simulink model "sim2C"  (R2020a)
settings: Solver=ode15s  StartTime=0.0  StopTime=tsim  RelTol=1e-3
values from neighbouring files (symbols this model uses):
  d0 = 0    [run2C.m]    (also in Main.m = [Fh, Tcin, Thin]; Main_OL.m = [Fh, Tcin, Thin]; runTestCalcBlk.m = [Fh, Tcin, Thin]; runTransf.m = [Fh; Tcin; U0; Ffeed0; m0; Tfeed0])
  df = 0    [run2C.m]
  h0 = [LC1max ; LC1min; LC2max; LC2min; LC3max;LC3min ]    [run2C.m]
  hf = h0    [run2C.m]
  hmax = [2.3; 2.8; 3.2]    [run2C.m]
  Kc = 1./k.*1./(tauC+theta)    [run2C.m]    (also in Main.m = 1/k*tau/(tauC+theta); runTransf.m = 1/kM(i)*tau(i)/(tauCM(i)+theta(i)); runTransfOL.m = 1/kM(i)*tau(i)/(tauCM(i)+theta(i)))
  KI = Kc./tauI    [run2C.m]    (also in Main.m = Kp/tauIv; Main_OL.m = 1; runTransf.m = 1/kS(i)*1/tauCS(i); runTransfOL.m = 1/kS(i)*1/tauCS(i))
  nd = length(d0)    [run2C.m]    (also in Main.m = size(d0,2); Main_OL.m = size(d0,2); runTestCalcBlk.m = size(d0,2); runTransf.m = size(d0,1))
  np = length(param)    [run2C.m]    (also in runH2Psim.m; Main.m = size(p,2); Main_OL.m = size(p,2); runTestCalcBlk.m = size(p,2))
  nu = length(z0)    [run2C.m]    (also in runH2Psim.m = length(u0); Main.m = 1; Main_OL.m = 1; runTestCalcBlk.m = 1)
  nx = length(x0)    [run2C.m]    (also in H2P_Turbine_driven.m = param(end); runTD.m; H2P_Boiler_driven.m = param(end); runBD.m)
  param = [A; Cv; DP; rho; N]    [run2C.m]    (also in runTD.m = [Tref;TrefB;dHvap;cpg;cpW;cpSt;R;Mwt;     T0;TG0;ME;pC;     ; runBD.m = [Tref;TrefB;dHvap;cpg;cpW;cpSt;R;Mwt;          T0;TG0;ME;pC;; runFP.m = [Tref;TrefB;dHvap;cpg;cpW;cpSt;R;Mwt;          T0;TG0;ME;pC;; runFPV2.m = [Tref;TrefB;dHvap;cpg;cpW;cpSt;R;Mwt;          T0;TG0;ME;pC;)
  tauT = tauI./2    [run2C.m]
  td = 0    [run2C.m]
  th = ones(6,1)    [run2C.m]
  tz0OP = [10; tBend]    [run2C.m]
  tz1OP = [10; tBend]    [run2C.m]
  tz2OP = [10; tBend]    [run2C.m]
  tz3OP = [10; tBend]    [run2C.m]
  u0 = [z0(1); z0(2); z0(2); z0(3); z0(3); z0(4)]    [run2C.m]    (also in runH2Psim.m = [mG0;zV0;mP0;mB0;mA0]; calcblock.m = p(2); testfun.m = 5; u_function.m = 5)
  x0 = [hH; hH; hH].*hmax    [run2C.m]    (also in runTD.m = [TE0;TD0;TSh0;MD0; MSh0;w0;TA0;0;0;0;0;0;0;0;0;0]; runBD.m = [TE0;TD0;TSh0;MD0; MSh0;w0;TA0;0;0;0;0;0;0;0;0;0]; runFP.m = [TE0;TD0;TSh0;MD0; MSh0;w0;TA0;0;0;0;0;0;0;0]; runFPV2.m = [TE0;TD0;TSh0;MD0; MSh0;w0;TA0;0;0;0;0;0;0;0])
  zOP = z0.*[0.5; 1; 1; 1]    [run2C.m]
  zOP0 = [1;1;1;1]    [run2C.m]
undefined symbols (not defined in the file or in its folder): TanksODE

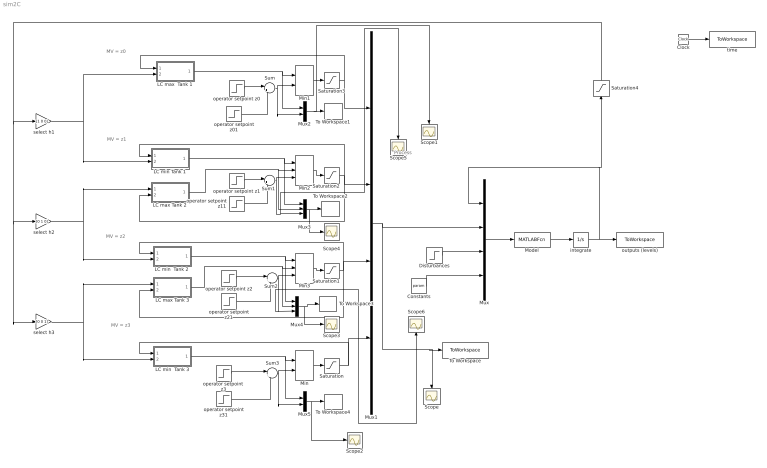
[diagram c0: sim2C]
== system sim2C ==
  note: MV = z3
  note: MV = z2
  note: MV = z1
  note: MV = z0
  note: Process
  Clock : Clock
  Constants : Constant  Value=param
  Disturbances : Step  Time=td  Before=d0  After=df  SampleTime=0
  LC max  Tank 1 : Subsystem
  LC max Tank 2 : Subsystem
  LC max Tank 3 : Subsystem
  "LC min  Tank 2 " : Subsystem
  LC min  Tank 3 : Subsystem
  LC min Tank 1 : Subsystem
  Min : MinMax  Inputs=2
  Min1 : MinMax  Inputs=2
  Min2 : MinMax  Inputs=3
  Min3 : MinMax  Inputs=3
  Model : MATLABFcn  MATLABFcn=TanksODE(u(1:nx),u(nx+1:nx+nu),u(nx+nu+1:nx+nu+nd),u(nx+nu+nd+1:nx+nu+nd+np))  OutputDimensions=nx
  Mux : Mux
  Mux1 : Mux
  Mux2 : Mux  Inputs=2
  Mux3 : Mux  Inputs=3
  Mux4 : Mux  Inputs=3
  Mux5 : Mux  Inputs=2
  Saturation{,1..3} (4 alike) : Saturate  UpperLimit=1  LowerLimit=0
  Saturation4 : Saturate  UpperLimit=hmax  LowerLimit=0
  Scope{,1..6} (7 alike) : Scope
  Sum{,1..3} (4 alike) : Sum  Inputs=|++
  To Workspace : ToWorkspace  VariableName=u2C  SampleTime=-1
  To Workspace1 : ToWorkspace  VariableName=u02C  SampleTime=-1
  To Workspace2 : ToWorkspace  VariableName=u12C  SampleTime=-1
  To Workspace3 : ToWorkspace  VariableName=u22C  SampleTime=-1
  To Workspace4 : ToWorkspace  VariableName=u32C  SampleTime=-1
  integrate : Integrator  InitialCondition=x0
  operator setpoint  z3 : Step  Time=tz3OP(1)  Before=zOP0(4)  After=zOP(4)  SampleTime=0
  operator setpoint z0 : Step  Time=tz0OP(1)  Before=zOP0(1)  After=zOP(1)  SampleTime=0
  operator setpoint z01 : Step  Time=tz0OP(2)  After=zOP0(1)-zOP(1)  SampleTime=0
  operator setpoint z1 : Step  Time=tz1OP(1)  Before=zOP0(2)  After=zOP(2)  SampleTime=0
  operator setpoint z11 : Step  Time=tz1OP(2)  After=zOP0(2)-zOP(2)  SampleTime=0
  operator setpoint z2 : Step  Time=tz2OP(1)  Before=zOP0(3)  After=zOP(3)  SampleTime=0
  operator setpoint z21 : Step  Time=tz2OP(2)  After=zOP0(3)-zOP(3)  SampleTime=0
  operator setpoint z31 : Step  Time=tz3OP(2)  After=zOP0(4)-zOP(4)  SampleTime=0
  outputs (levels) : ToWorkspace  VariableName=y2C  SampleTime=-1
  select h1 : Gain  Gain=[1 0 0]  Multiplication=Matrix(K*u)
  select h2 : Gain  Gain=[0 1 0]  Multiplication=Matrix(K*u)
  select h3 : Gain  Gain=[0 0 1]  Multiplication=Matrix(K*u)
  time : ToWorkspace  VariableName=t2C  SampleTime=-1
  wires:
  Clock/1 -> time/1
  Mux/1 -> Model/1
  Model/1 -> integrate/1
  integrate/1 -> outputs (levels)/1, Mux/1, Saturation4/1
  Constants/1 -> Mux/4
  Disturbances/1 -> Mux/3
  Mux1/1 -> Scope/1, To Workspace/1, Mux/2
  Saturation3/1 -> Mux1/1, LC max  Tank 1/1(In2)
  Saturation2/1 -> LC max Tank 2/2(In1), Mux1/2, LC min Tank 1/1(In2)
  Saturation1/1 -> LC max Tank 3/2(In1), Mux1/3, "LC min  Tank 2 "/1(In2)
  Saturation/1 -> Mux1/4, LC min  Tank 3/1(In2)
  Min/1 -> Saturation/1
  Min2/1 -> Saturation2/1
  Min3/1 -> Saturation1/1
  Min1/1 -> Saturation3/1
  LC max  Tank 1/1(Outport) -> Mux2/1, Min1/1
  operator setpoint z0/1 -> Sum/1
  LC max Tank 2/1(Outport) -> Mux3/2, Min2/2
  operator setpoint  z3/1 -> Sum3/1
  select h1/1 -> LC max  Tank 1/2(In1), LC min Tank 1/2(In1)
  LC min Tank 1/1(Outport) -> Mux3/1, Min2/1
  select h2/1 -> LC max Tank 2/1(In2), "LC min  Tank 2 "/2(In1)
  "LC min  Tank 2 "/1(Outport) -> Mux4/1, Min3/1
  LC max Tank 3/1(Outport) -> Mux4/2, Min3/2
  operator setpoint z2/1 -> Sum2/1
  operator setpoint z1/1 -> Sum1/1
  select h3/1 -> LC max Tank 3/1(In2), LC min  Tank 3/2(In1)
  Saturation4/1 -> select h3/1, select h2/1, select h1/1
  Sum/1 -> Mux2/2, Min1/2
  operator setpoint z01/1 -> Sum/2
  Sum1/1 -> Scope5/1, Mux3/3, Min2/3
  operator setpoint z11/1 -> Sum1/2
  Sum2/1 -> Scope6/1, Mux4/3, Min3/3
  operator setpoint z21/1 -> Sum2/2
  Sum3/1 -> Mux5/2, Min/2
  operator setpoint z31/1 -> Sum3/2
  LC min  Tank 3/1(Outport) -> Mux5/1, Min/1
  Mux2/1 -> Scope1/1, To Workspace1/1
  Mux3/1 -> Scope4/1, To Workspace2/1
  Mux4/1 -> Scope3/1, To Workspace3/1
  Mux5/1 -> Scope2/1, To Workspace4/1

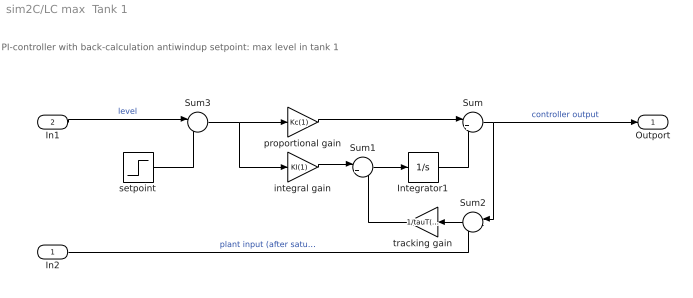
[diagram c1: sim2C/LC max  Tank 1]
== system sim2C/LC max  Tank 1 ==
  note: PI-controller with back-calculation antiwindup setpoint: max level in tank 1
  In2 : Inport
  In1 : Inport  Port=2
  Integrator1 : Integrator  InitialCondition=u0(1)
  Sum : Sum  Inputs=|++
  Sum1 : Sum  Inputs=|++
  Sum2 : Sum  Inputs=|-+
  Sum3 : Sum  Inputs=|-+
  integral gain : Gain  Gain=KI(1)  Multiplication=Matrix(K*u)
  proportional gain : Gain  Gain=Kc(1)  Multiplication=Matrix(K*u)
  setpoint : Step  Time=th(1)  Before=h0(1)  After=hf(1)  SampleTime=0
  tracking gain : Gain  Gain=1/tauT(1)  Multiplication=Matrix(K*u)
  Outport : Outport
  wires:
  In1/1 -> Sum3/1  "level"
  proportional gain/1 -> Sum/1
  Integrator1/1 -> Sum/2
  setpoint/1 -> Sum3/2
  Sum3/1 -> integral gain/1, proportional gain/1
  Sum2/1 -> tracking gain/1
  integral gain/1 -> Sum1/1
  Sum1/1 -> Integrator1/1
  tracking gain/1 -> Sum1/2
  Sum/1 -> Outport/1, Sum2/1  "controller output"
  In2/1 -> Sum2/2  "plant input (after saturation block)"

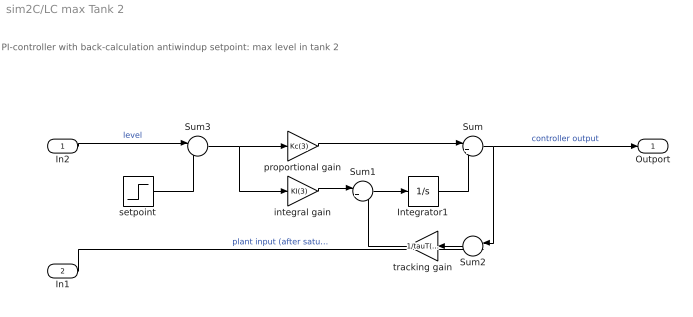
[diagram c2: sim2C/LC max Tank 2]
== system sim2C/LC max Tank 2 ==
  note: PI-controller with back-calculation antiwindup setpoint: max level in tank 2
  In2 : Inport
  In1 : Inport  Port=2
  Integrator1 : Integrator  InitialCondition=u0(3)
  Sum : Sum  Inputs=|++
  Sum1 : Sum  Inputs=|++
  Sum2 : Sum  Inputs=|-+
  Sum3 : Sum  Inputs=|-+
  integral gain : Gain  Gain=KI(3)  Multiplication=Matrix(K*u)
  proportional gain : Gain  Gain=Kc(3)  Multiplication=Matrix(K*u)
  setpoint : Step  Time=th(3)  Before=h0(3)  After=hf(3)  SampleTime=0
  tracking gain : Gain  Gain=1/tauT(3)  Multiplication=Matrix(K*u)
  Outport : Outport
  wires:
  In1/1 -> Sum2/2  "plant input (after saturation)"
  Sum/1 -> Sum2/1, Outport/1  "controller output"
  tracking gain/1 -> Sum1/2
  Sum1/1 -> Integrator1/1
  integral gain/1 -> Sum1/1
  Sum2/1 -> tracking gain/1
  Sum3/1 -> proportional gain/1, integral gain/1
  setpoint/1 -> Sum3/2
  Integrator1/1 -> Sum/2
  proportional gain/1 -> Sum/1
  In2/1 -> Sum3/1  "level"

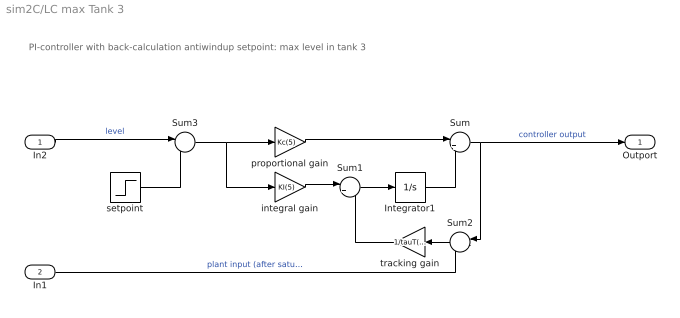
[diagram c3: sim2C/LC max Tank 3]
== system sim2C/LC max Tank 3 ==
  note: PI-controller with back-calculation antiwindup setpoint: max level in tank 3
  In2 : Inport
  In1 : Inport  Port=2
  Integrator1 : Integrator  InitialCondition=u0(5)
  Sum : Sum  Inputs=|++
  Sum1 : Sum  Inputs=|++
  Sum2 : Sum  Inputs=|-+
  Sum3 : Sum  Inputs=|-+
  integral gain : Gain  Gain=KI(5)  Multiplication=Matrix(K*u)
  proportional gain : Gain  Gain=Kc(5)  Multiplication=Matrix(K*u)
  setpoint : Step  Time=th(5)  Before=h0(5)  After=hf(5)  SampleTime=0
  tracking gain : Gain  Gain=1/tauT(5)  Multiplication=Matrix(K*u)
  Outport : Outport
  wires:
  In2/1 -> Sum3/1  "level"
  proportional gain/1 -> Sum/1
  Integrator1/1 -> Sum/2
  setpoint/1 -> Sum3/2
  Sum3/1 -> integral gain/1, proportional gain/1
  Sum2/1 -> tracking gain/1
  integral gain/1 -> Sum1/1
  Sum1/1 -> Integrator1/1
  tracking gain/1 -> Sum1/2
  Sum/1 -> Outport/1, Sum2/1  "controller output"
  In1/1 -> Sum2/2  "plant input (after saturation)"

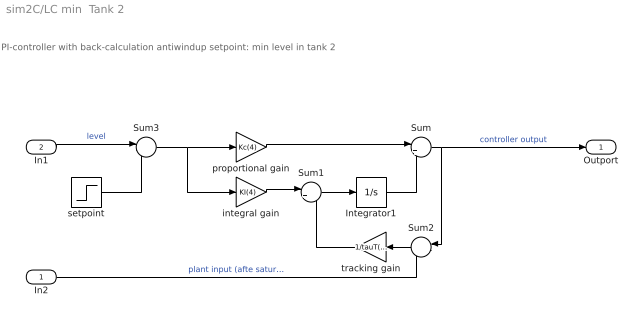
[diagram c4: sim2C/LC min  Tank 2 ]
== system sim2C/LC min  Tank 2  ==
  note: PI-controller with back-calculation antiwindup setpoint: min level in tank 2
  In2 : Inport
  In1 : Inport  Port=2
  Integrator1 : Integrator  InitialCondition=u0(4)
  Sum : Sum  Inputs=|++
  Sum1 : Sum  Inputs=|++
  Sum2 : Sum  Inputs=|-+
  Sum3 : Sum  Inputs=|-+
  integral gain : Gain  Gain=KI(4)  Multiplication=Matrix(K*u)
  proportional gain : Gain  Gain=Kc(4)  Multiplication=Matrix(K*u)
  setpoint : Step  Time=th(4)  Before=h0(4)  After=hf(4)  SampleTime=0
  tracking gain : Gain  Gain=1/tauT(4)  Multiplication=Matrix(K*u)
  Outport : Outport
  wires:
  In1/1 -> Sum3/1  "level"
  proportional gain/1 -> Sum/1
  Integrator1/1 -> Sum/2
  setpoint/1 -> Sum3/2
  Sum3/1 -> integral gain/1, proportional gain/1
  Sum2/1 -> tracking gain/1
  integral gain/1 -> Sum1/1
  Sum1/1 -> Integrator1/1
  tracking gain/1 -> Sum1/2
  Sum/1 -> Outport/1, Sum2/1  "controller output"
  In2/1 -> Sum2/2  "plant input (afte saturation)"

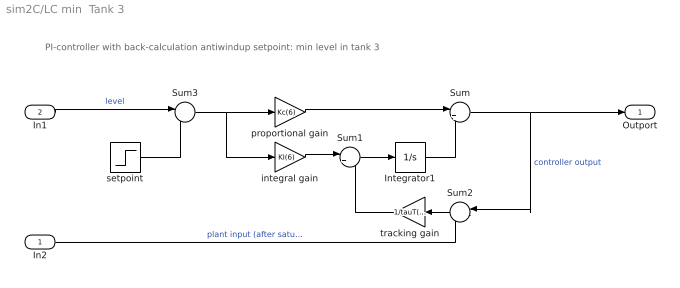
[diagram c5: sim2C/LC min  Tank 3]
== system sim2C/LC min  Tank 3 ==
  note: PI-controller with back-calculation antiwindup setpoint: min level in tank 3
  In2 : Inport
  In1 : Inport  Port=2
  Integrator1 : Integrator  InitialCondition=u0(6)
  Sum : Sum  Inputs=|++
  Sum1 : Sum  Inputs=|++
  Sum2 : Sum  Inputs=|-+
  Sum3 : Sum  Inputs=|-+
  integral gain : Gain  Gain=KI(6)  Multiplication=Matrix(K*u)
  proportional gain : Gain  Gain=Kc(6)  Multiplication=Matrix(K*u)
  setpoint : Step  Time=th(6)  Before=h0(6)  After=hf(6)  SampleTime=0
  tracking gain : Gain  Gain=1/tauT(6)  Multiplication=Matrix(K*u)
  Outport : Outport
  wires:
  In1/1 -> Sum3/1  "level"
  proportional gain/1 -> Sum/1
  Integrator1/1 -> Sum/2
  setpoint/1 -> Sum3/2
  Sum3/1 -> integral gain/1, proportional gain/1
  Sum2/1 -> tracking gain/1
  integral gain/1 -> Sum1/1
  Sum1/1 -> Integrator1/1
  tracking gain/1 -> Sum1/2
  Sum/1 -> Outport/1, Sum2/1  "controller output"
  In2/1 -> Sum2/2  "plant input (after saturation)"

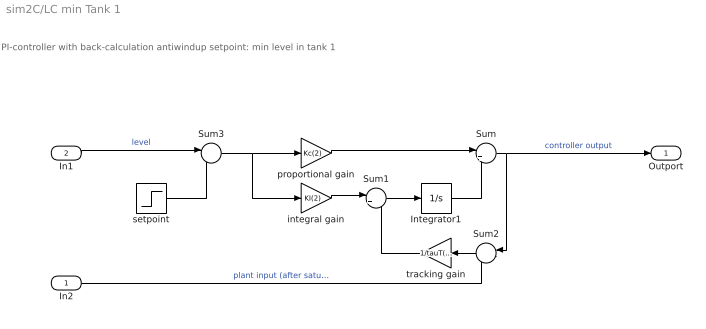
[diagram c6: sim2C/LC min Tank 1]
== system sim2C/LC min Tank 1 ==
  note: PI-controller with back-calculation antiwindup setpoint: min level in tank 1
  In2 : Inport
  In1 : Inport  Port=2
  Integrator1 : Integrator  InitialCondition=u0(2)
  Sum : Sum  Inputs=|++
  Sum1 : Sum  Inputs=|++
  Sum2 : Sum  Inputs=|-+
  Sum3 : Sum  Inputs=|-+
  integral gain : Gain  Gain=KI(2)  Multiplication=Matrix(K*u)
  proportional gain : Gain  Gain=Kc(2)  Multiplication=Matrix(K*u)
  setpoint : Step  Time=th(2)  Before=h0(2)  After=hf(2)  SampleTime=0
  tracking gain : Gain  Gain=1/tauT(2)  Multiplication=Matrix(K*u)
  Outport : Outport
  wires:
  In1/1 -> Sum3/1  "level"
  proportional gain/1 -> Sum/1
  Integrator1/1 -> Sum/2
  setpoint/1 -> Sum3/2
  Sum3/1 -> integral gain/1, proportional gain/1
  Sum2/1 -> tracking gain/1
  integral gain/1 -> Sum1/1
  Sum1/1 -> Integrator1/1
  tracking gain/1 -> Sum1/2
  Sum/1 -> Outport/1, Sum2/1  "controller output"
  In2/1 -> Sum2/2  "plant input (after saturation)"
